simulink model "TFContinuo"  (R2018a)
settings: Solver=VariableStepAuto  StartTime=0.0  StopTime=3000  RelTol=1e-3
undefined symbols (not defined in the file): b2e2, b861, bb0aaedc, sdiscope, TFContinuo

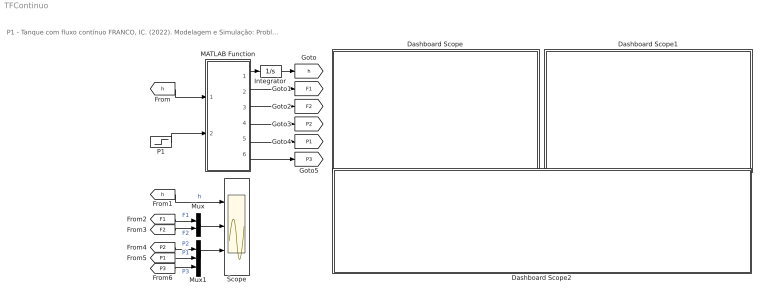
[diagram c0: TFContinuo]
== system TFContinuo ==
  note: P1 - Tanque com fluxo contínuo FRANCO, IC. (2022). Modelagem e Simulação: Problemas Típicos da Engenharia Química para Simulação e Análise. NOTAS DE AULA INOVADORAS. The Journal of Engineering and Exact Sciences. Material Complementar.
  Dashboard Scope : Subsystem  DialogController=hmiCreateDDGDialog  IsWebBlock=on  mask(MWDashboardBlock){webBlockId=bb0aaedc-e254-47b2-83d2-97ef23d4ce5b, webBlockType=sdiscope, ShowInitialText=on, HMISrcModelName=TFContinuo}
      mask prompts: webBlockId "WebBlock Id"; webBlockType "WebBlock Type"; HMISrcModelName "Source Model"
      mask help: SimulinkHMI:dialogs:HMIScopeDialogDesc
  Dashboard Scope1 : Subsystem  DialogController=hmiCreateDDGDialog  IsWebBlock=on  mask(MWDashboardBlock){webBlockId=9562f2ce-4f72-4572-9857-123cd0054c03, webBlockType=sdiscope, ShowInitialText=on, HMISrcModelName=TFContinuo}
      mask prompts: webBlockId "WebBlock Id"; webBlockType "WebBlock Type"; HMISrcModelName "Source Model"
      mask help: SimulinkHMI:dialogs:HMIScopeDialogDesc
  Dashboard Scope2 : Subsystem  DialogController=hmiCreateDDGDialog  IsWebBlock=on  mask(MWDashboardBlock){webBlockId=7037474d-b2e2-42b8-b861-2872c06be339, webBlockType=sdiscope, ShowInitialText=on, HMISrcModelName=TFContinuo}
      mask prompts: webBlockId "WebBlock Id"; webBlockType "WebBlock Type"; HMISrcModelName "Source Model"
      mask help: SimulinkHMI:dialogs:HMIScopeDialogDesc
  Integrator : Integrator  InitialCondition=3  LimitOutput=on  UpperSaturationLimit=4  LowerSaturationLimit=0
  MATLAB Function : MATLAB Function  TreatAsAtomicUnit=on
  Mux : Mux  Inputs=2
  Mux1 : Mux  Inputs=3
  P1 : Step  Time=1000  Before=110  After=110  SampleTime=0
  Scope : Scope  NumInputPorts=3
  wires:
  MATLAB Function/1(dh) -> Integrator/1
  Integrator/1 -> [h]
  MATLAB Function/2(F1) -> [F1]
  MATLAB Function/3(F2) -> [F2]
  [h] -> MATLAB Function/1(h)
  P1/1 -> MATLAB Function/2("P1 ")
  [h] -> Scope/1  "h"
  [F1] -> Mux/1  "F1"
  [F2] -> Mux/2  "F2"
  Mux/1 -> Scope/2
  MATLAB Function/4(P2) -> [P2]
  MATLAB Function/5(P1) -> [P1]
  MATLAB Function/6(P3) -> [P3]
  [P2] -> Mux1/1  "P2"
  [P1] -> Mux1/2  "P1"
  [P3] -> Mux1/3  "P3"
  Mux1/1 -> Scope/3

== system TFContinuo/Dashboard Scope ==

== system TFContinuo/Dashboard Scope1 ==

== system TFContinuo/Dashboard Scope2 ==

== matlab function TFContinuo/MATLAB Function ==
function [dh,F1,F2,P2,P1,P3] = fcn(h,P1)
%% dados do processo
A    =    1.000;
g    =    9.810;
hmax =    4.000;
k1   =    0.001;
k2   =    0.001;
P0   =  101.325;
P3   =  101.325;
TG0  =  330.000;
rho  = 1000.000;
gamma=    1.410;

%% equações auxiliares
P2=P0+(rho*g*h)/1000;

% condicional para evitar valor negativo
if P2>P1
   P2=P1;
end

F1=k1*sqrt(P1-P2);
F2=k2*sqrt(P2-P3);

%% modelos matemáticos
dh = (F1-F2)/A;
end
